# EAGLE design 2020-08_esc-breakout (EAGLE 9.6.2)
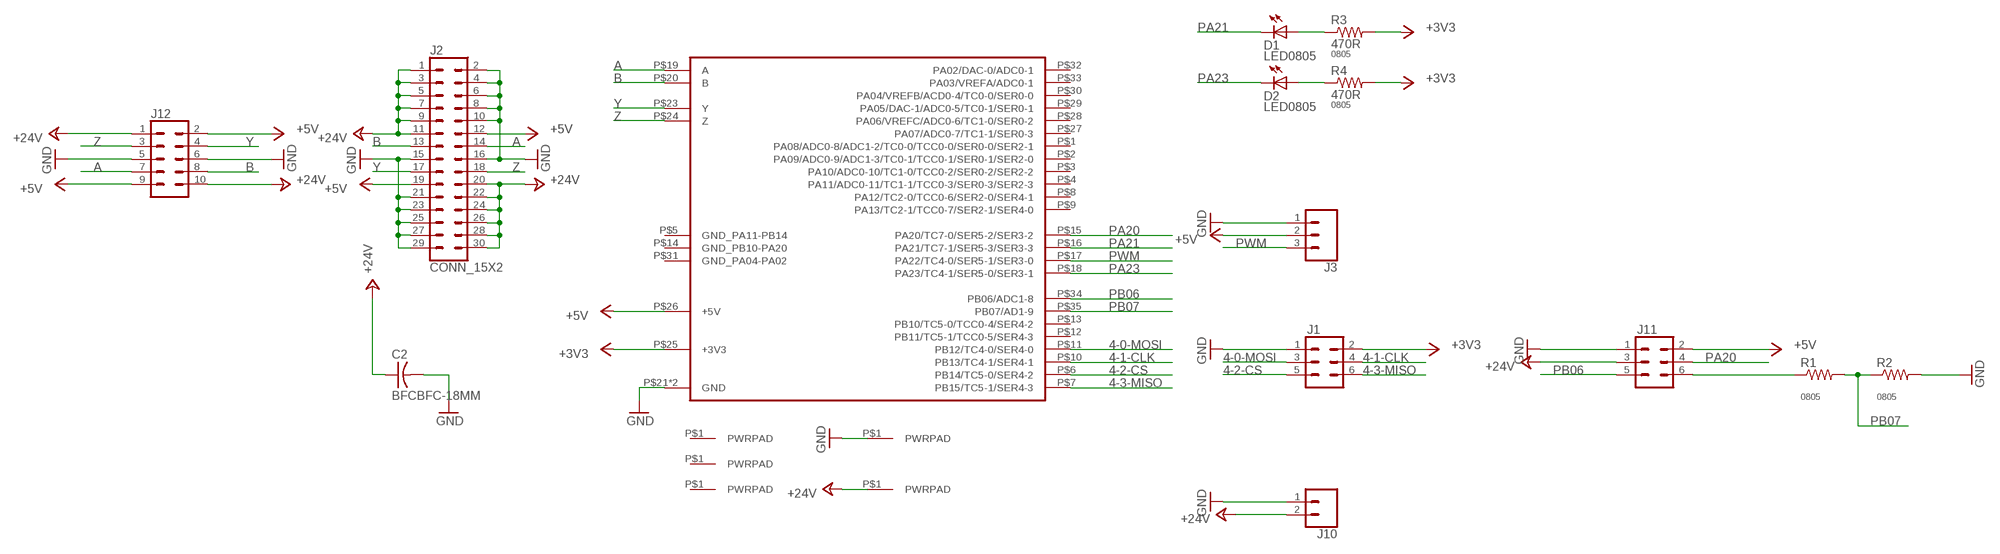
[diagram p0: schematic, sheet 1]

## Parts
C2  BFCBFC-18MM  [BFC-18MM-7-5MM]
D1  LED0805  [LED0805]
D2  LED0805  [LED0805]
J1  CONN_03X2SHROUD  [2X3-SHROUDED]
J2  CONN_15X2  [2X15-SHROUDED]
J3  CONN_03LOCK_NO_SILK  [1X03_LOCK_NO_SILK]
J4  PWRPADM3-SKINNY  [PWRPAD_3-25MM-SKINNY]
J5  PWRPADM3-SKINNY  [PWRPAD_3-25MM-SKINNY]
J6  PWRPADM3-SKINNY  [PWRPAD_3-25MM-SKINNY]
J7  PWRPADSOLDER  [SOLDER_ON]
J8  PWRPADSOLDER  [SOLDER_ON]
J10  CONN_02LOCK  [1X02_LOCK]
J11  CONN_03X2SHROUD  [2X3-SHROUDED]
J12  CONN_05X2SHD_LOCK_LATCH  [2X5-SHROUDED_LOCK_LATCH]
R1  RESISTOR0805-RES  [0805]
R2  RESISTOR0805-RES  [0805]
R3  470R  RESISTOR0805-RES  [0805]
R4  470R  RESISTOR0805-RES  [0805]
U1  UCBUS_MODULE  [UCBUS_MODULE]

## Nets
4-0-MOSI: J1.3 U1.P$11(PB12/TC4-0/SER4-0)
4-1-CLK: J1.4 U1.P$10(PB13/TC4-1/SER4-1)
4-2-CS: J1.5 U1.P$6(PB14/TC5-0/SER4-2)
4-3-MISO: J1.6 U1.P$7(PB15/TC5-1/SER4-3)
+3V3: J1.2 R3.2 R4.2 U1.P$25(+3V3)
+5V: J2.12 J2.19 J3.2 J11.2 J12.2 J12.9 U1.P$26(+5V)
+24V: C2.P$2 J2.1 J2.3 J2.5 J2.7 J2.9 J2.11 J2.20 J2.22 J2.24 J2.26 J2.28 J2.30 J8.P$1(PWRPAD) J10.2 J11.3 J12.1 J12.10
A: J2.14 J12.7 U1.P$19(A)
B: J2.13 J12.8 U1.P$20(B)
GND: C2.P$1 J1.1 J2.2 J2.4 J2.6 J2.8 J2.10 J2.15 J2.16 J2.21 J2.23 J2.25 J2.27 J2.29 J3.1 J7.P$1(PWRPAD) J10.1 J11.1 J12.5 J12.6 R2.2 U1.P$21(GND) U1.P$22(GND)
N$1: D1.1(A) R3.1
N$3: J11.6 R1.1
N$4: D2.1(A) R4.1
PA20: J11.4 U1.P$15(PA20/TC7-0/SER5-2/SER3-2)
PA21: D1.2(C) U1.P$16(PA21/TC7-1/SER5-3/SER3-3)
PA23: D2.2(C) U1.P$18(PA23/TC4-1/SER5-0/SER3-1)
PB06: J11.5 U1.P$34(PB06/ADC1-8)
PB07: R1.2 R2.1 U1.P$35(PB07/AD1-9)
PWM: J3.3 U1.P$17(PA22/TC4-0/SER5-1/SER3-0)
Y: J2.17 J12.4 U1.P$23(Y)
Z: J2.18 J12.3 U1.P$24(Z)
Unconnected: J4.P$1(PWRPAD) J5.P$1(PWRPAD) J6.P$1(PWRPAD) U1.P$1(PA08/ADC0-8/ADC1-2/TC0-0/TCC0-0/SER0-0/SER2-1) U1.P$2(PA09/ADC0-9/ADC1-3/TC0-1/TCC0-1/SER0-1/SER2-0) U1.P$3(PA10/ADC0-10/TC1-0/TCC0-2/SER0-2/SER2-2) U1.P$4(PA11/ADC0-11/TC1-1/TCC0-3/SER0-3/SER2-3) U1.P$5(GND_PA11-PB14) U1.P$8(PA12/TC2-0/TCC0-6/SER2-0/SER4-1) U1.P$9(PA13/TC2-1/TCC0-7/SER2-1/SER4-0) U1.P$12(PB11/TC5-1/TCC0-5/SER4-3) U1.P$13(PB10/TC5-0/TCC0-4/SER4-2) U1.P$14(GND_PB10-PA20) U1.P$27(PA07/ADC0-7/TC1-1/SER0-3) U1.P$28(PA06/VREFC/ADC0-6/TC1-0/SER0-2) U1.P$29(PA05/DAC-1/ADC0-5/TC0-1/SER0-1) U1.P$30(PA04/VREFB/ACD0-4/TC0-0/SER0-0) U1.P$31(GND_PA04-PA02) U1.P$32(PA02/DAC-0/ADC0-1) U1.P$33(PA03/VREFA/ADC0-1)

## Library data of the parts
C2 = power:BFC
D1 D2 = lights:LED: LED
J1 J11 = SparkFun-Connectors:CONN_03X2: Multi connection point. Often used as Generic Header-pin footprint for 0.1 inch spaced/style header connections You can populate with any combo of single row headers, but if you'd like an exact match, check these: Header - 2x3 (Male, 0.1") (PRT-12807) Header - 2x3 (Female, 0.1") (PRT-13010) 2x3 Pin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; PROD_ID: CONN-10681; SF_ID: PRT_10877
J2 = SparkFun-Connectors:CONN_15X2
J3 = SparkFun-Connectors:CONN_03: Multi connection point. Often used as Generic Header-pin footprint for 0.1 inch spaced/style header connections On any of the 0.1 inch spaced packages, you can populate with these: Break Away Headers - Straight (PRT-00116) Break Away Male Headers - Right Angle (PRT-00553) Female Headers (PRT-00115)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
J4-J8 = connector:PWRPAD
J10 = SparkFun-Connectors:CONN_02: Multi connection point. Often used as Generic Header-pin footprint for 0.1 inch spaced/style header connections
J12 = SparkFun-Connectors:CONN_05X2: Multi connection point. Often used as Generic Header-pin footprint for 0.1 inch spaced/style header connections For AVR SPI programming port, see special device with nice symbol: "AVR_SPI_PROG_5x2.dev" You can populate with any combo of single row headers, but if you'd like an exact match, check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
R1-R4 = passives:RESISTOR: Resistor; PACKAGE: 0805
U1 = connector:UCBUS_MODULE

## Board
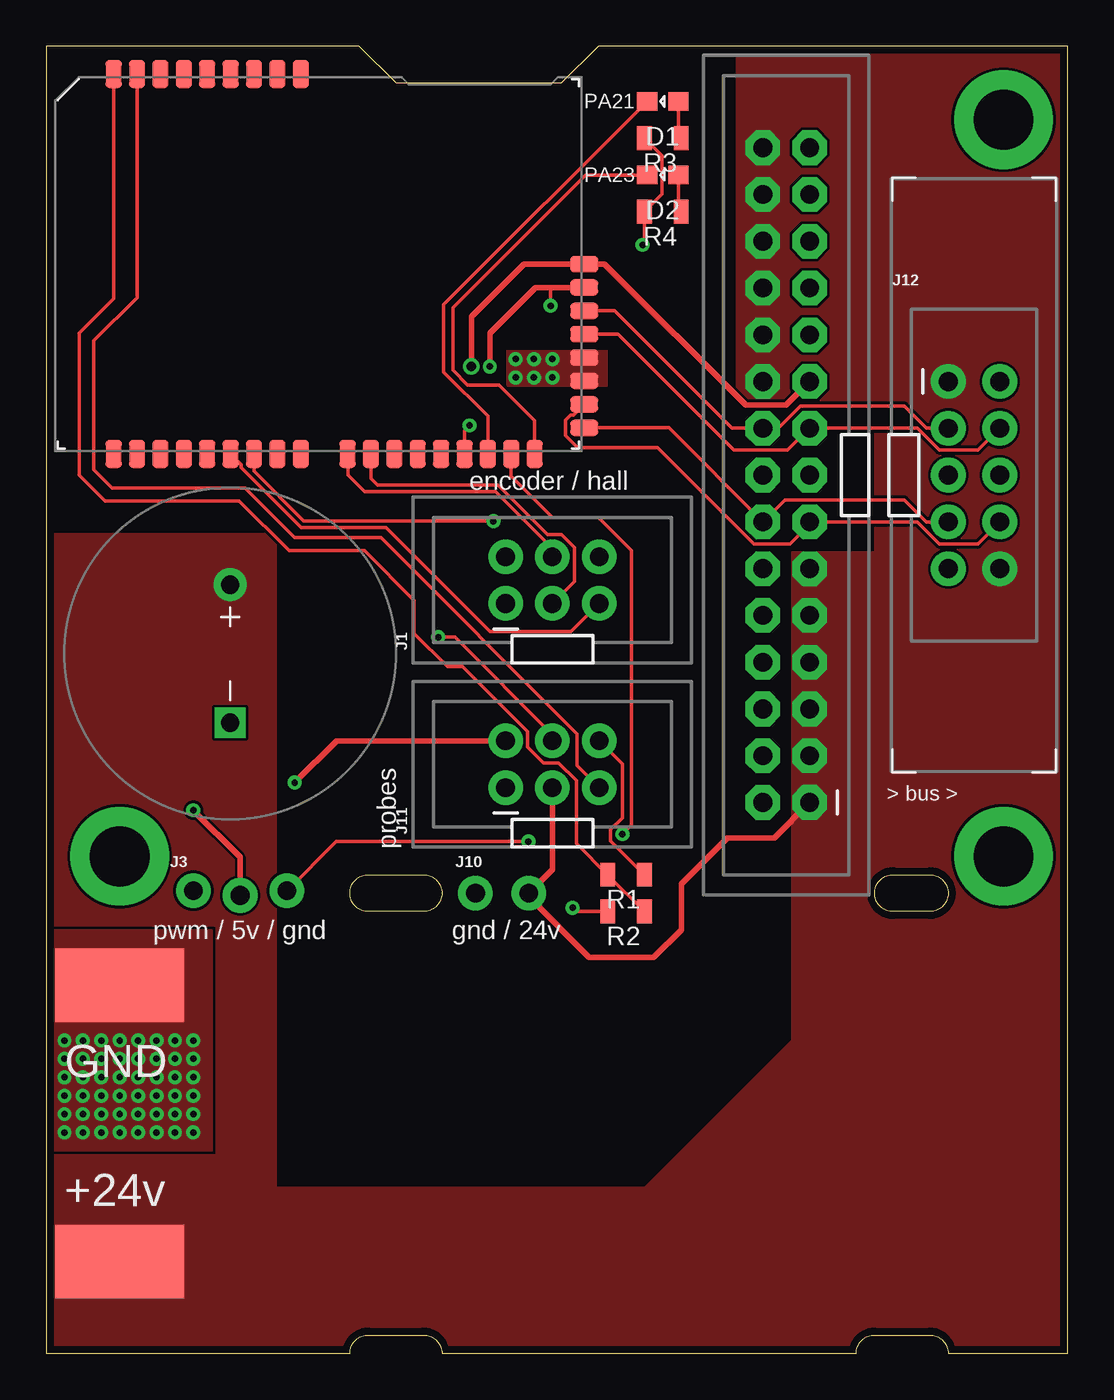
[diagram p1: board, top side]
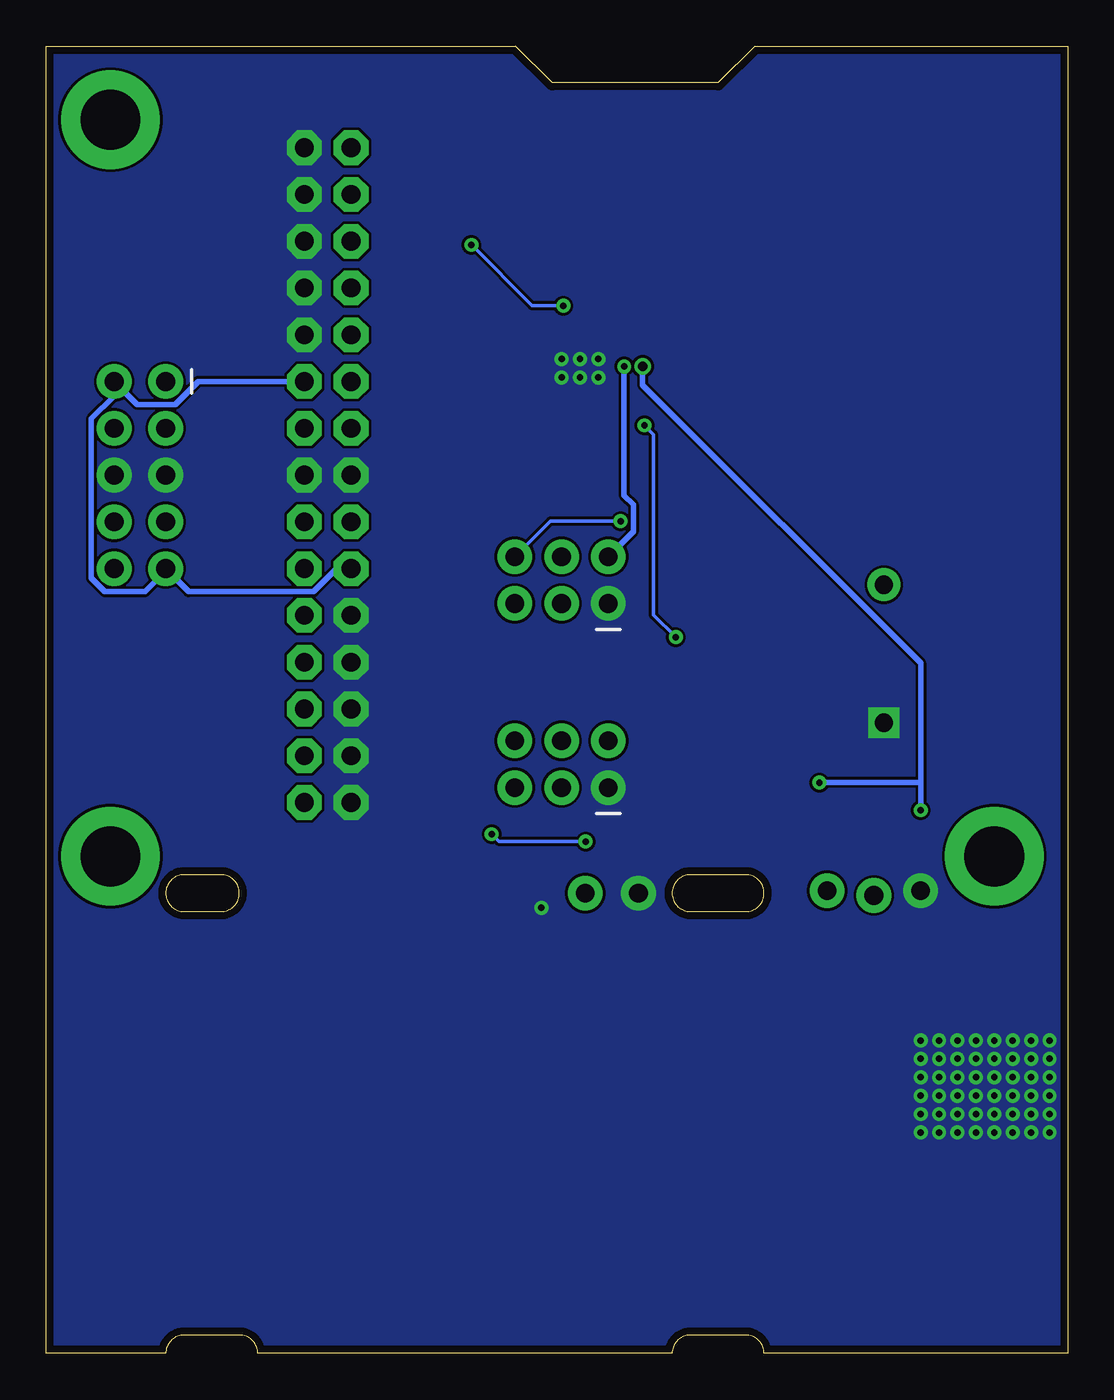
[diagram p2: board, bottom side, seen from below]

Size 55.5 x 71 mm. Coordinates in mm from the lower left corner, seen from the top.
Outline: 0,0 16.5,0 arc-90 17.5,1 20.5,1 arc-90 21.5,0 44,0 arc-90 45,1 48,1 arc-90 49,0 55.5,0 55.5,71 30,71 28,69 19,69 17,71 0,71 0,0
Outline: 16.5,25 arc-90 17.5,26 20.5,26 arc-90 21.5,25 arc-90 20.5,24 17.5,24 arc-90 16.5,25
Outline: 45,25 arc-90 46,26 48,26 arc-90 49,25 arc-90 48,24 46,24 arc-90 45,25
Copper layers (1*16): Top 0.035mm / dielectric 1.5mm / Bottom 0.035mm
Design rules "default *": minimum track width 6mil, minimum drill 0.35mm, track to track 6mil, track to pad 6mil, pad to pad 6mil, via to via 6mil, smd to smd 6mil, copper to edge 16mil, drill to drill 6mil, minimum pad ring 10mil, minimum via ring 8mil, stop-mask expansion 4mil, vias tented up to drill 30mil, thermal gap 10mil

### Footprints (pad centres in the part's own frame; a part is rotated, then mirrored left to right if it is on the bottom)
BFC-18MM-7-5MM = drill 1 pad 1.676 square: P$1 -3.75,0 | drill 1 pad 1.778: P$2 3.75,0
LED0805 = smd 1.1 x 1: 1 -0.85,0; 2 0.85,0
2X3-SHROUDED = drill 1.016 pad 1.88: 1 -1.27,2.54; 2 1.27,2.54; 3 -1.27,0; 4 1.27,0; 5 -1.27,-2.54; 6 1.27,-2.54
2X15-SHROUDED = drill 1.016 pad 1.88 octagon: 1 -1.27,17.78; 2 1.27,17.78; 3 -1.27,15.24; 4 1.27,15.24; 5 -1.27,12.7; 6 1.27,12.7; 7 -1.27,10.16; 8 1.27,10.16; 9 -1.27,7.62; 10 1.27,7.62; 11 -1.27,5.08; 12 1.27,5.08; 13 -1.27,2.54; 14 1.27,2.54; 15 -1.27,0; 16 1.27,0; 17 -1.27,-2.54; 18 1.27,-2.54; 19 -1.27,-5.08; 20 1.27,-5.08; 21 -1.27,-7.62; 22 1.27,-7.62; 23 -1.27,-10.16; 24 1.27,-10.16; 25 -1.27,-12.7; 26 1.27,-12.7; 27 -1.27,-15.24; 28 1.27,-15.24; 29 -1.27,-17.78; 30 1.27,-17.78
1X03_LOCK_NO_SILK = drill 1.016 pad 1.88: 1 0,0.127; 2 2.54,-0.127; 3 5.08,0.127
PWRPAD_3-25MM-SKINNY = drill 3.25 pad 5.35: P$1 0,0
SOLDER_ON = smd 4 x 7: P$1 0,0
1X02_LOCK = drill 1.016 pad 1.88: 1 -0.178,0; 2 2.718,0
2X5-SHROUDED_LOCK_LATCH = drill 1.016 pad 1.88: 1 -1.397,5.08; 2 1.397,5.08; 3 -1.397,2.54; 4 1.397,2.54; 5 -1.397,0; 6 1.397,0; 7 -1.397,-2.54; 8 1.397,-2.54; 9 -1.397,-5.08; 10 1.397,-5.08
0805 = smd 0.8 x 1.3: 1 -1,0; 2 1,0
UCBUS_MODULE = smd 0.889 x 1.524: P$1 3.175,-0.152; P$2 4.445,-0.152; P$3 5.715,-0.152; P$4 6.985,-0.152; P$5 8.255,-0.152; P$6 9.525,-0.152; P$7 10.795,-0.152; P$8 12.065,-0.152; P$9 13.335,-0.152; P$10 15.875,-0.152; P$11 17.145,-0.152; P$12 18.415,-0.152; P$13 19.685,-0.152; P$14 20.955,-0.152; P$15 22.225,-0.152; P$16 23.495,-0.152; P$17 24.765,-0.152; P$18 26.035,-0.152; P$27 13.335,20.472; P$28 12.065,20.472; P$29 10.795,20.472; P$30 9.525,20.472; P$31 8.255,20.472; P$32 6.985,20.472; P$33 5.715,20.472; P$34 4.445,20.472; P$35 3.175,20.472 | smd 1.524 x 0.889: P$19 28.727,1.27; P$20 28.727,2.54; P$21 28.727,3.81; P$22 28.727,5.08; P$23 28.727,6.35; P$24 28.727,7.62; P$25 28.727,8.89; P$26 28.727,10.16

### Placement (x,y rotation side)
C2  10,38 90 top
D1  33.5,68 180 top
D2  33.5,64 180 top
J1  27.5,42 90 top
J2  40.2,47.7 180 top
J3  8,25 0 top
J4  4,27 0 top
J5  52,67 0 top
J6  52,27 0 top
J7  4,20 90 top
J8  4,5 90 top
J10  23.5,25 0 top
J11  27.5,32 90 top
J12  50.4,47.7 0 top
R1  31.5,26 180 top
R2  31.5,24 180 top
R3  33.5,66 180 top
R4  33.5,62 180 top
U1  0.5,49 0 top

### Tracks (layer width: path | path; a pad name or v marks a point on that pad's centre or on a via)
4-0-MOSI
  Top 0.203: U1.P$11 17.64,47.51 18,47.16 24.55,47.16 27.24,44.46 27.99,44.46 28.69,43.76 28.69,41.92 J1.3
4-1-CLK
  Top 0.203: U1.P$10 16.4,48.82 16.4,47.7 17.3,46.8 24.4,46.8 27.5,43.7 J1.4
4-2-CS
  Top 0.203: U1.P$6 10.6,48.28 10.6,48.1 13.85,44.84 18.46,44.84 24.1,39.2 28.51,39.2 J1.5
4-3-MISO  (via drill 0.35)
  Top 0.203: U1.P$7 11.29,47.91 14,45.2 v24.3,45.2
  Bottom 0.203: v24.3,45.2 28.11,45.2 J1.6
+3V3  (via drill 0.35)
  Top 0.203: R3.2 33.45,65.05 33.45,62.95 R4.2 32.5,60.3 v32.4,60.2 | v27.4,56.9 27.4,57.89
  Top 0.305: U1.P$25 27.4,57.89 26.59,57.89 24.1,55.4 v24.1,53.6
  Bottom 0.203: v32.4,60.2 29.1,56.9 v27.4,56.9
  Bottom 0.305: v24.1,53.6 24.1,46.6 23.6,46.1 23.6,44.63 J1.2
+5V  (via drill 0.35, 0.5)
  Top 0.305: v23.1,53.6 23.1,56.3 25.96,59.16 U1.P$26 30.34,59.16 38,51.5 40.19,51.5 J2.19 | v8,29.5 10.54,26.96 J3.2 | v13.5,31 15.77,33.27 J11.2
  Bottom 0.305: J2.19 47.24,52.78 48.49,51.53 50.55,51.53 J12.2 51.8,52 53.04,50.76 53.04,42.1 52.31,41.38 50.12,41.38 48.94,42.56 | J2.12 39.71,42.62 40.95,41.38 47.76,41.38 48.94,42.56 | 48.94,42.56 J12.9 | v23.1,53.6 23.1,52.6 8,37.5 8,31 | 8,31 v8,29.5 | 8,31 v13.5,31
+24V
  Top 0.305: J2.1 39.55,28 37,28 34.5,25.5 34.5,23 33,21.5 29.5,21.5 26.22,24.78 J10.2 27.5,26.28 J11.3
  pour Top (rank 2, no thermals): 37.5,73 37.5,51.5 45,51.5 45,43.5 40.5,43.5 40.5,17 32.5,9 12.5,9 12.5,44 12,44.5 -2,44.5 -2,-2 57.5,-2 57.5,73
A
  Top 0.203: J12.7 47.82,45.16 46.62,46.35 40.12,46.35 J2.14 33.82,50.27 U1.P$19
B
  Top 0.203: J2.13 41.6,45.16 | 41.6,45.16 47.31,45.16 48.51,43.97 50.6,43.97 J12.8 | U1.P$20 28.66,50.97 28.49,50.97 28.21,50.69 28.21,49.85 28.86,49.2 33.2,49.2 38.44,43.97 40.41,43.97 41.6,45.16
GND  (via drill 0.35)
  Top 0.203: R2.2 28.8,24 v28.6,24.2
  other vias: 1,17 2,17 3,17 4,17 5,17 6,17 7,17 8,17 1,16 2,16 3,16 4,16 5,16 6,16 7,16 8,16 1,15 2,15 3,15 4,15 5,15 6,15 7,15 8,15 1,14 2,14 3,14 4,14 5,14 6,14 7,14 8,14 1,13 2,13 3,13 4,13 5,13 6,13 7,13 8,13 1,12 2,12 3,12 4,12 5,12 6,12 7,12 8,12 26.5,54 26.5,53 27.5,53 27.5,54 25.5,54 25.5,53
  pour Bottom (no thermals): -1,72 56.5,72 56.5,-1 -1,-1
  pour Top: -3,23 9,23 9,11 -3,11
  pour Top (rank 2, no thermals): 30.5,54.5 25,54.5 25,52.5 30.5,52.5
N$1
  Top 0.203: R3.1 34.35,66.15 D1.1
N$3
  Top 0.203: J11.6 31.3,32.01 31.3,29.09 30.67,28.46 30.67,27.83 R1.1
N$4
  Top 0.203: R4.1 34.35,62.15 D2.1
PA20  (via drill 0.35)
  Top 0.203: U1.P$15 22.73,50.12 v23,50.4 | J11.4 27.5,33.6 22.2,38.9 v21.3,38.9
  Bottom 0.203: v23,50.4 22.5,49.9 22.5,40.1 v21.3,38.9
PA21
  Top 0.203: D1.2 21.6,56.95 21.6,53.3 24,50.91 U1.P$16
PA23
  Top 0.203: U1.P$18 26.54,50.66 24.6,52.6 22.9,52.6 22.1,53.4 22.1,56.8 29.3,64 D2.2
PB06
  Top 0.203: J11.5 28.85,31.92 28.85,33.65 18.2,44.3 13.5,44.3 10.8,47 3.6,47 2.6,48 2.6,55 4.95,57.34 U1.P$34
PB07
  Top 0.203: R2.1 R1.2 28.8,27.7 28.8,31.12 27.84,32.08 27.01,32.08 26.15,32.93 26.15,33.76 22.62,37.3 21.8,37.3 20,39.1 20,40.9 17.3,43.6 13.2,43.6 10.5,46.3 3.2,46.3 1.8,47.7 1.8,55.4 3.67,57.27 U1.P$35
PWM  (via drill 0.35)
  Top 0.203: U1.P$17 25.27,47.63 27.5,45.4 30,45.4 31.8,43.6 31.8,28.7 v31.3,28.2 | v26.2,27.8 15.75,27.8 J3.3
  Bottom 0.203: v31.3,28.2 30.9,27.8 v26.2,27.8
Y
  Top 0.203: J12.4 50.6,49.05 48.51,49.05 47.31,50.24 J2.17 40.28,49.05 37.35,49.05 31.05,55.35 U1.P$23
Z
  Top 0.203: J12.3 47.82,50.24 46.62,51.43 40.98,51.43 39.78,50.24 39,50.24 J2.18 37.26,50.24 30.88,56.62 U1.P$24

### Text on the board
tPlace: PA21 | PA23 | encoder / hall | probes | > bus > | pwm / 5v / gnd | gnd / 24v | GND | +24v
